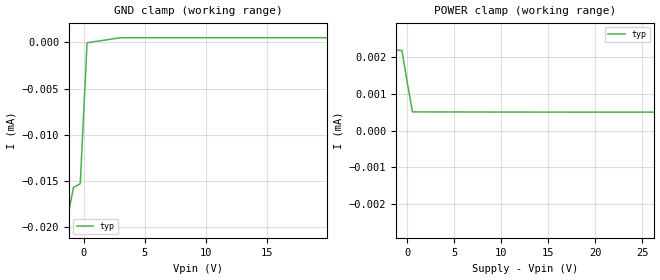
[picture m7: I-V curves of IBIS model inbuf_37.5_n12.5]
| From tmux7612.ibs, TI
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| inbuf_37.5_n12.5
[Model]   inbuf_37.5_n12.5
Model_type   Input
Vinl = 0.8
Vinh = 1.3
|   typ   min   max
C_comp   1.008417e-12   NA   NA
[Voltage Range]   37.5_12.5   NA   NA
[Temperature Range]   27   NA   NA
[Power Clamp Reference]   37.5_12.5   NA   NA
[GND Clamp Reference]   0   NA   NA
[GND Clamp]
|   Voltage   I(typ)   I(min)   I(max)
-17.5V    -3.924A    NA         NA
-13.61V   -45.51mA   NA         NA
-13.06V   -18.2uA    NA         NA
-12.5V    -17.91uA   NA         NA
-2.5V     -16.8uA    NA         NA
-1.944V   -25.48uA   NA         NA
-1.389V   -19.4uA    NA         NA
-833.3mV  -15.68uA   NA         NA
-277.8mV  -15.27uA   NA         NA
277.8mV   -55.39nA   NA         NA
36.94V    508.1nA    NA         NA
37.5V     1.32uA     NA         NA
[POWER Clamp]
|   Voltage   I(typ)   I(min)   I(max)
-5V       247.8uA    NA         NA
-4.444V   8.278uA    NA         NA
-3.889V   2.293uA    NA         NA
-555.6mV  2.175uA    NA         NA
0V        1.32uA     NA         NA
555.6mV   508.1nA    NA         NA
34.44V    499nA      NA         NA
37.22V    -55.39nA   NA         NA
37.78V    -15.27uA   NA         NA
50V       -17.91uA   NA         NA
